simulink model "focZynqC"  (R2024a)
settings: Solver=ode45  StartTime=0.0  StopTime=10.0  RelTol=1e-3  EnableMultiTasking=on
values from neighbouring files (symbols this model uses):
  dataRange = Rotor velocity
                        radian/sec
                        800.0
                        -800.0
                    
                
                
                    
                        Phase current
                        Ampere
                        12.0
                        -12.0    [focZynqData.sldd]
  paramEncoderCalibrationDuration = 0.2
                
                    
                        Auto
                        
                        
                        -1.0
                        Simulink
                        Parameter
                        Default
                        
                            
                                0    [focZynqData.sldd]
  paramEncoderCalibrationMaxError = 0.0012566370614359172
                
                    
                        Auto
                        
                        
                        -1.0
                        Simulink
                        Parameter
                        Default
                        
                            
                                0    [focZynqData.sldd]
  paramEncoderCalibrationVoltage = 2.0
                
                    
                        Auto
                        
                        
                        -1.0
                        Simulink
                        Parameter
                        Default
                        
                            
                                0    [focZynqData.sldd]
  paramEncoderRotorPositionAtZeroCount = 0.0
                
                    
                        Auto
                        
                        
                        -1.0
                        Simulink
                        Parameter
                        Default
                        
                            
                                0    [focZynqData.sldd]
  paramOpenLoopVelocityAcceleration = 40.0
                
                    
                        Auto
                        
                        
                        -1.0
                        Simulink
                        Parameter
                        Default
                        
                            
                                0    [focZynqData.sldd]
  paramOpenLoopVelocityToVoltsBias = 0.4
                
                    
                        Auto
                        
                        
                        -1.0
                        Simulink
                        Parameter
                        Default
                        
                            
                                0    [focZynqData.sldd]
  paramOpenLoopVelocityToVoltsScalar = 0.04
                
                    
                        Auto
                        
                        
                        -1.0
                        Simulink
                        Parameter
                        Default
                        
                            
                                0    [focZynqData.sldd]
  paramVelocityControlI = 0.1
                
                    
                        Auto
                        
                        
                        -1.0
                        Simulink
                        Parameter
                        Default
                        
                            
                                0    [focZynqData.sldd]
  paramVelocityControlP = 0.02
                
                    
                        Auto
                        
                        
                        -1.0
                        Simulink
                        Parameter
                        Default
                        
                            
                                0    [focZynqData.sldd]
  paramVelocityControlSatCurrent = 4.0
                
                    
                        Auto
                        
                        
                        -1.0
                        Simulink
                        Parameter
                        Default
                        
                            
                                0    [focZynqData.sldd]
  pmsm = Dyno 1: BLY172D-24V-4000 Anaheim Automation
                BLY172D-24V-4000 Anaheim Automation
Phase A leads B leads C for counterclockwise rotation
-----------------------------------------------------
Phase A = Yellow
Phase B = Red
Phase C = Black
                
                    
                        Watt
                        Volt
                        rad/sec    [focZynqData.sldd]
  sampleTime = 4.0E-5
                0.001
                0.001
                4.0E-5
                2.0E-8
                4.0E-5
                0.001
                2.0E-8
                2.0E-8
                2.0E-8    [focZynqData.sldd]
libraries: simulink x2

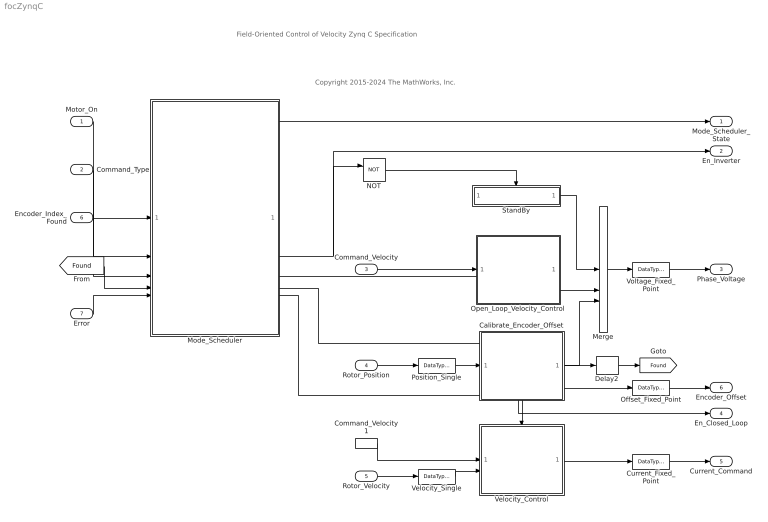
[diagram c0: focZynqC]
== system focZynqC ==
  note: Copyright 2015-2024 The MathWorks, Inc.
  note: Field-Oriented Control of Velocity Zynq C Specification
  Motor_On : Inport  OutDataTypeStr=boolean
  Command_Type : Inport  Port=2  OutDataTypeStr=Enum: commandTypeEnum
  Command_Velocity : Inport  Port=3
  Rotor_Position : Inport  Port=4  OutMin=0  OutMax=2*pi  OutDataTypeStr=fixdt(1,16,12)  SampleTime=sampleTime.VelocityControl
  Rotor_Velocity : Inport  Port=5  OutMin=dataRange.RotorVelocity.Min  OutMax=dataRange.RotorVelocity.Max  OutDataTypeStr=fixdt(1,16,5)
  Encoder_Index_Found : Inport  Port=6  OutDataTypeStr=boolean
  Error : Inport  Port=7  OutDataTypeStr=boolean
  Calibrate_Encoder_Offset : Subsystem
  Command_Velocity1 : InportShadow  Port=3
  Current_Fixed_Point : DataTypeConversion  OutMin=dataRange.PhaseCurrent.Min  OutMax=dataRange.PhaseCurrent.Max  OutDataTypeStr=fixdt(1,16,11)
  Delay2 : Delay  DelayLength=1
  Merge : Merge  Inputs=3
  Mode_Scheduler : Stateflow chart  TreatAsAtomicUnit=on
  NOT : Logic  Operator=NOT  IconShape=distinctive  AllPortsSameDT=off  OutDataTypeStr=boolean
  Offset_Fixed_Point : DataTypeConversion  OutMin=0  OutMax=2*pi  OutDataTypeStr=fixdt(1,16,12)
  Open_Loop_Velocity_Control : Subsystem  TreatAsAtomicUnit=on
  Position_Single : DataTypeConversion  OutDataTypeStr=single
  StandBy : Subsystem  Description=Stand By mode for controller outputs constant phase voltages.  TreatAsAtomicUnit=on
  Velocity_Control : Subsystem
  Velocity_Single : DataTypeConversion  OutDataTypeStr=single
  Voltage_Fixed_Point : DataTypeConversion  OutMin=dataRange.DqVoltage.Min  OutMax=dataRange.DqVoltage.Max  OutDataTypeStr=fixdt(1,16,11)
  Mode_Scheduler_State : Outport  VectorParamsAs1DForOutWhenUnconnected=off
  En_Inverter : Outport  Port=2  VectorParamsAs1DForOutWhenUnconnected=off
  Phase_Voltage : Outport  Port=3  VectorParamsAs1DForOutWhenUnconnected=off
  En_Closed_Loop : Outport  Port=4  VectorParamsAs1DForOutWhenUnconnected=off
  Current_Command : Outport  Port=5  VectorParamsAs1DForOutWhenUnconnected=off
  Encoder_Offset : Outport  Port=6  VectorParamsAs1DForOutWhenUnconnected=off
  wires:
  Rotor_Velocity/1 -> Velocity_Single/1
  Encoder_Index_Found/1 -> Mode_Scheduler/3(encoderIndexFound)
  Command_Velocity1/1 -> Velocity_Control/1(Velocity_Command)
  Command_Velocity/1 -> Open_Loop_Velocity_Control/1(Velocity_Command)
  [Found] -> Mode_Scheduler/4(encoderOffsetFound)
  Mode_Scheduler/4(" calibrateEncoder") -> Calibrate_Encoder_Offset/Enable
  Mode_Scheduler/1(mode) -> Mode_Scheduler_State/1
  Command_Type/1 -> Mode_Scheduler/2(commandType)
  Delay2/1 -> [Found]
  Error/1 -> Mode_Scheduler/5(error)
  Rotor_Position/1 -> Position_Single/1
  Calibrate_Encoder_Offset/3(Position_At_Zero_Count) -> Offset_Fixed_Point/1
  Calibrate_Encoder_Offset/2(Position_At_Zero_Count_Valid) -> Delay2/1
  Merge/1 -> Voltage_Fixed_Point/1
  Open_Loop_Velocity_Control/1(Phase_Voltage) -> Merge/2
  Calibrate_Encoder_Offset/1(Phase_Voltage) -> Merge/3
  Velocity_Control/1(Q_Current_Command) -> Current_Fixed_Point/1
  Motor_On/1 -> Mode_Scheduler/1(motorOn)
  Mode_Scheduler/3(" openLoop") -> Open_Loop_Velocity_Control/Enable
  Mode_Scheduler/5(" closedLoop") -> Velocity_Control/Enable, En_Closed_Loop/1
  Mode_Scheduler/2(" enableInverter") -> NOT/1, En_Inverter/1
  NOT/1 -> StandBy/Enable
  StandBy/1(Phase Voltage) -> Merge/1
  Voltage_Fixed_Point/1 -> Phase_Voltage/1
  Current_Fixed_Point/1 -> Current_Command/1
  Position_Single/1 -> Calibrate_Encoder_Offset/1(Rotor_Position)
  Velocity_Single/1 -> Velocity_Control/2(Velocity_Measured)
  Offset_Fixed_Point/1 -> Encoder_Offset/1

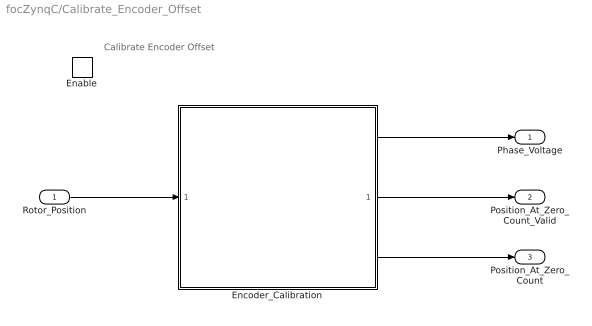
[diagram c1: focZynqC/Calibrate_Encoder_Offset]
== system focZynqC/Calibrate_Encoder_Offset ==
  note: Calibrate Encoder Offset
  Rotor_Position : Inport  PortDimensions=1  Interpolate=off
  Enable : EnablePort  StatesWhenEnabling=reset
  Encoder_Calibration : Subsystem
  Phase_Voltage : Outport  PortDimensions=3  InitialOutput=0  VectorParamsAs1DForOutWhenUnconnected=off
  Position_At_Zero_Count_Valid : Outport  Port=2  InitialOutput=0  VectorParamsAs1DForOutWhenUnconnected=off
  Position_At_Zero_Count : Outport  Port=3  InitialOutput=paramEncoderRotorPositionAtZeroCount  VectorParamsAs1DForOutWhenUnconnected=off
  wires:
  Encoder_Calibration/3(Position_At_Zero_Count) -> Position_At_Zero_Count/1
  Encoder_Calibration/2(Position_Valid) -> Position_At_Zero_Count_Valid/1
  Encoder_Calibration/1(Phase_Voltage) -> Phase_Voltage/1
  Rotor_Position/1 -> Encoder_Calibration/1(Rotor_Position)

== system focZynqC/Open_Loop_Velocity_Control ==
  note: Open Loop Velocity Control
  Velocity_Command : Inport
  Enable : EnablePort  StatesWhenEnabling=reset
  Open_Loop_Velocity_Control : Subsystem
  Phase_Voltage : Outport  VectorParamsAs1DForOutWhenUnconnected=off
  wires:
  Open_Loop_Velocity_Control/1(Phase_Voltage) -> Phase_Voltage/1  "phaseVoltage"
  Velocity_Command/1 -> Open_Loop_Velocity_Control/1(Velocity_Command)

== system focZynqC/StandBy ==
  note: Disabled
  Enable : EnablePort
  Constant : Constant  Value=[0 0 0]  OutDataTypeStr=Inherit: Inherit via back propagation
  Phase Voltage : Outport  InitialOutput=[0 0 0]  VectorParamsAs1DForOutWhenUnconnected=off
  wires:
  Constant/1 -> Phase Voltage/1

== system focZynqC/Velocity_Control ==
  note: Velocity Control
  Velocity_Command : Inport
  Velocity_Measured : Inport  Port=2
  Enable : EnablePort  StatesWhenEnabling=reset
  Velocity_Control : Subsystem
  Q_Current_Command : Outport  InitialOutput=0  VectorParamsAs1DForOutWhenUnconnected=off
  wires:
  Velocity_Command/1 -> Velocity_Control/1(Velocity_Command)
  Velocity_Measured/1 -> Velocity_Control/2(Velocity_Measured)  "rotorVelocity"
  Velocity_Control/1(Current) -> Q_Current_Command/1  "qCurrentCommand"

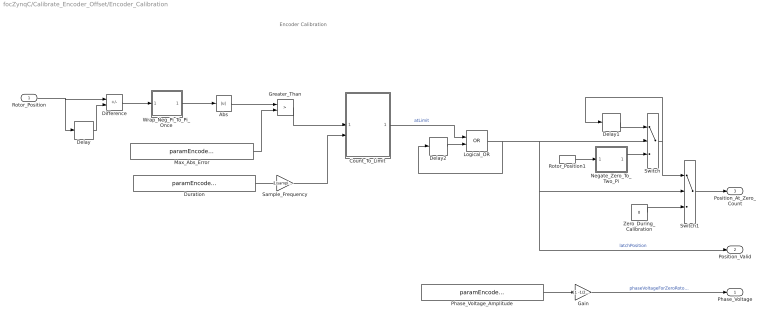
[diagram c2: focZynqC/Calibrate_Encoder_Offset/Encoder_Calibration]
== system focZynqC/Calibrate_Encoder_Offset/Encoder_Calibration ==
  note: Encoder Calibration
  Rotor_Position : Inport  OutMin=0  OutMax=2*pi  PortDimensions=1  SampleTime=sampleTime.EncoderCalibration  Interpolate=off
  Abs : Abs
  Count_To_Limit : Subsystem
  Delay : Delay  DelayLength=1
  Delay1 : Delay  DelayLength=1  InitialCondition=0
  Delay2 : Delay  DelayLength=1  InitialCondition=0
  Difference : Sum  Inputs=+-
  Duration : Constant  Value=paramEncoderCalibrationDuration  OutDataTypeStr=Inherit: Inherit via back propagation  SampleTime=-1
  Gain : Gain  Gain=[1 -1/2 -1/2]
  Greater_Than : RelationalOperator  Operator=>  OutDataTypeStr=boolean
  Logical_OR : Logic  Operator=OR  IconShape=distinctive  AllPortsSameDT=off  OutDataTypeStr=boolean
  Max_Abs_Error : Constant  Value=paramEncoderCalibrationMaxError  OutDataTypeStr=Inherit: Inherit via back propagation  SampleTime=-1
  Negate_Zero_To_Two_Pi : Subsystem
  Phase_Voltage_Amplitude : Constant  Value=paramEncoderCalibrationVoltage  OutDataTypeStr=Inherit: Inherit via back propagation  SampleTime=-1
  Rotor_Position1 : InportShadow  OutMin=0  OutMax=2*pi  PortDimensions=1  SampleTime=sampleTime.EncoderCalibration  Interpolate=off
  Sample_Frequency : Gain  Gain=1/sampleTime.EncoderCalibration
  Switch : Switch  Criteria=u2 ~= 0  Threshold=1
  Switch1 : Switch  Threshold=1
  Wrap_Neg_Pi_To_Pi_Once : Subsystem
  Zero_During_Calibration : Constant  Value=0  OutDataTypeStr=Inherit: Inherit via back propagation
  Phase_Voltage : Outport  SampleTime=sampleTime.EncoderCalibration  InitialOutput=0  VectorParamsAs1DForOutWhenUnconnected=off
  Position_Valid : Outport  Port=2  SampleTime=sampleTime.EncoderCalibration  InitialOutput=0  VectorParamsAs1DForOutWhenUnconnected=off
  Position_At_Zero_Count : Outport  Port=3  SampleTime=sampleTime.EncoderCalibration  InitialOutput=0  VectorParamsAs1DForOutWhenUnconnected=off
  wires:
  Greater_Than/1 -> Count_To_Limit/1(Reset)
  Gain/1 -> Phase_Voltage/1  "phaseVoltageForZeroRotorPosition"
  Phase_Voltage_Amplitude/1 -> Gain/1
  Duration/1 -> Sample_Frequency/1
  Difference/1 -> Wrap_Neg_Pi_To_Pi_Once/1(Position)
  Wrap_Neg_Pi_To_Pi_Once/1(Wrap) -> Abs/1
  Switch1/1 -> Position_At_Zero_Count/1
  Abs/1 -> Greater_Than/1
  Max_Abs_Error/1 -> Greater_Than/2
  Zero_During_Calibration/1 -> Switch1/3
  Logical_OR/1 -> Delay2/1, Position_Valid/1, Switch1/2, Switch/2  "latchPosition"
  Rotor_Position/1 -> Delay/1, Difference/1
  Switch/1 -> Switch1/1, Delay1/1
  Delay/1 -> Difference/2
  Rotor_Position1/1 -> Negate_Zero_To_Two_Pi/1(In)
  Delay1/1 -> Switch/1
  Negate_Zero_To_Two_Pi/1(Out) -> Switch/3
  Sample_Frequency/1 -> Count_To_Limit/2(Limit)
  Count_To_Limit/1(At_Limit) -> Logical_OR/1  "atLimit"
  Delay2/1 -> Logical_OR/2

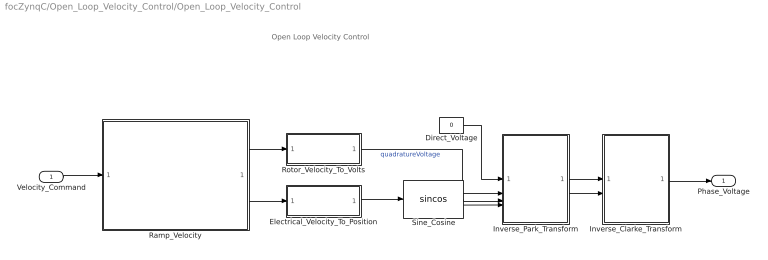
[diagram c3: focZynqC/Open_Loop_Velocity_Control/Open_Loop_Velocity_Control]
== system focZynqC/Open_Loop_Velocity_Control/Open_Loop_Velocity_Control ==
  note: Open Loop Velocity Control
  Velocity_Command : Inport  SampleTime=sampleTime.OpenLoopVelocityControl
  Direct_Voltage : Constant  Value=0  OutDataTypeStr=Inherit: Inherit via back propagation
  Electrical_Velocity_To_Position : Subsystem
  Inverse_Clarke_Transform : Subsystem  VariantControl=INVERSE_CLARKE_TRANSFORM
  Inverse_Park_Transform : Subsystem
  Ramp_Velocity : Subsystem
  Rotor_Velocity_To_Volts : Subsystem
  Sine_Cosine : Trigonometry  Operator=sincos
  Phase_Voltage : Outport  SampleTime=sampleTime.OpenLoopVelocityControl  VectorParamsAs1DForOutWhenUnconnected=off
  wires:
  Inverse_Clarke_Transform/1(ABC) -> Phase_Voltage/1
  Velocity_Command/1 -> Ramp_Velocity/1(Velocity_Command)
  Rotor_Velocity_To_Volts/1(V) -> Inverse_Park_Transform/2(Q)  "quadratureVoltage"
  Direct_Voltage/1 -> Inverse_Park_Transform/1(D)
  Inverse_Park_Transform/1(Alpha) -> Inverse_Clarke_Transform/1(Alpha)
  Inverse_Park_Transform/2(Beta) -> Inverse_Clarke_Transform/2(Beta)
  Ramp_Velocity/1(Rotor_Velocity) -> Rotor_Velocity_To_Volts/1(RV)
  Ramp_Velocity/2(Electrical_Velocity) -> Electrical_Velocity_To_Position/1(EV)
  Sine_Cosine/1 -> Inverse_Park_Transform/3(Sin_Coefficient1)
  Sine_Cosine/2 -> Inverse_Park_Transform/4(Cos_Coefficient1)
  Electrical_Velocity_To_Position/1(EP) -> Sine_Cosine/1

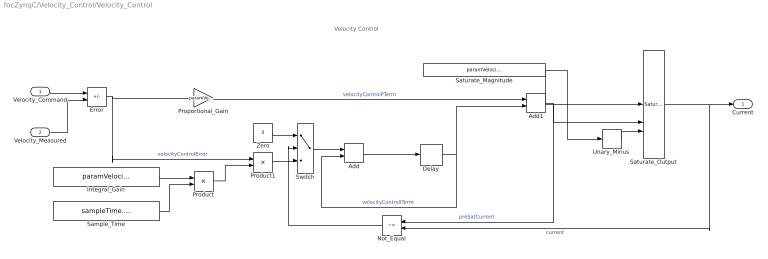
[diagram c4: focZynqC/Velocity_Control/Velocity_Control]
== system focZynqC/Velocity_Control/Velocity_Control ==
  note: Velocity Control
  Velocity_Command : Inport  SampleTime=sampleTime.VelocityControl
  Velocity_Measured : Inport  Port=2  SampleTime=sampleTime.VelocityControl
  Add : Sum
  Add1 : Sum
  Delay : Delay  DelayLength=1
  Error : Sum  Inputs=+-
  Integral_Gain : Constant  Value=paramVelocityControlI  OutDataTypeStr=Inherit: Inherit via back propagation
  Not_Equal : RelationalOperator  Operator=~=  OutDataTypeStr=boolean
  Product : Product
  Product1 : Product
  Proportional_Gain : Gain  Gain=paramVelocityControlP
  Sample_Time : Constant  Value=sampleTime.VelocityControl  OutDataTypeStr=Inherit: Inherit via back propagation
  Saturate_Magnitude : Constant  Value=paramVelocityControlSatCurrent  OutDataTypeStr=Inherit: Inherit via back propagation
  Saturate_Output : simulink/Discontinuities/Saturation Dynamic  OutMin=[]  OutMax=[]  OutDataTypeStr=Inherit: Same as second input  OutDataType=fixdt(1, 16)  OutScaling=2^-10  DoSatur=off
  Switch : Switch  Criteria=u2 ~= 0
  Unary_Minus : UnaryMinus
  Zero : Constant  Value=0  OutDataTypeStr=Inherit: Inherit via back propagation
  Current : Outport  SampleTime=sampleTime.VelocityControl  VectorParamsAs1DForOutWhenUnconnected=off
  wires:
  Add/1 -> Delay/1
  Product1/1 -> Switch/3
  Product/1 -> Product1/2
  Sample_Time/1 -> Product/2
  Integral_Gain/1 -> Product/1
  Unary_Minus/1 -> Saturate_Output/3
  Saturate_Magnitude/1 -> Unary_Minus/1, Saturate_Output/1
  Zero/1 -> Switch/1
  Switch/1 -> Add/1
  Not_Equal/1 -> Switch/2
  Saturate_Output/1 -> Not_Equal/2, Current/1  "current"
  Error/1 -> Product1/1, Proportional_Gain/1  "velocityControlError"
  Proportional_Gain/1 -> Add1/1  "velocityControlPTerm"
  Velocity_Command/1 -> Error/1
  Add1/1 -> Saturate_Output/2, Not_Equal/1  "preSatCurrent"
  Delay/1 -> Add1/2, Add/2  "velocityControlITerm"
  Velocity_Measured/1 -> Error/2

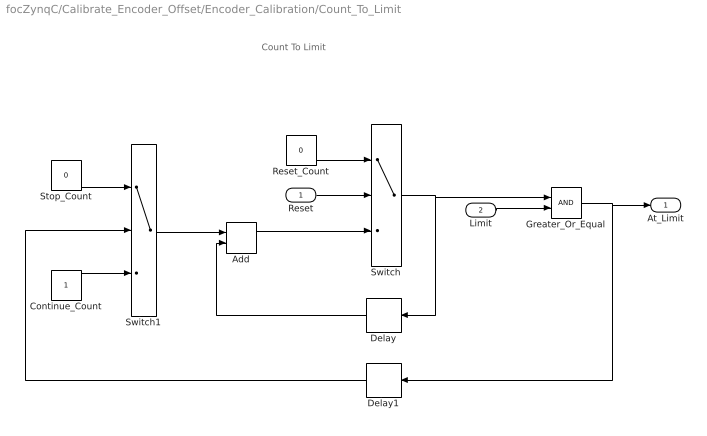
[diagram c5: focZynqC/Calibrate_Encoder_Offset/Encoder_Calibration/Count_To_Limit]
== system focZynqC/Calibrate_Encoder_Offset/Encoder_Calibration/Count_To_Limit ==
  note: Count To Limit
  Reset : Inport
  Limit : Inport  Port=2
  Add : Sum
  Continue_Count : Constant  OutDataTypeStr=Inherit: Inherit via back propagation
  Delay : Delay  DelayLength=1  InitialCondition=0
  Delay1 : Delay  DelayLength=1  InitialCondition=0
  Greater_Or_Equal : RelationalOperator  OutDataTypeStr=boolean
  Reset_Count : Constant  Value=0  OutDataTypeStr=Inherit: Inherit via back propagation
  Stop_Count : Constant  Value=0  OutDataTypeStr=Inherit: Inherit via back propagation
  Switch : Switch  Threshold=1
  Switch1 : Switch  Threshold=1
  At_Limit : Outport  VectorParamsAs1DForOutWhenUnconnected=off
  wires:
  Add/1 -> Switch/3
  Reset_Count/1 -> Switch/1
  Reset/1 -> Switch/2
  Delay/1 -> Add/2
  Greater_Or_Equal/1 -> At_Limit/1, Delay1/1
  Stop_Count/1 -> Switch1/1
  Switch/1 -> Greater_Or_Equal/1, Delay/1
  Continue_Count/1 -> Switch1/3
  Switch1/1 -> Add/1
  Limit/1 -> Greater_Or_Equal/2
  Delay1/1 -> Switch1/2

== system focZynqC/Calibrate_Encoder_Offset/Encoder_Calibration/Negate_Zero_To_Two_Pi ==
  note: Negate Zero To Two Pi
  In : Inport
  Input_Range : SignalSpecification  OutMin=0  OutMax=2*pi
  Subtract : Sum  Inputs=+-  OutDataTypeStr=Inherit: Inherit via back propagation
  Two_Pi : Constant  Value=2*pi  OutDataTypeStr=Inherit: Inherit via back propagation
  Out : Outport  VectorParamsAs1DForOutWhenUnconnected=off
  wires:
  Subtract/1 -> Out/1  "negativeIn"
  In/1 -> Input_Range/1
  Two_Pi/1 -> Subtract/1
  Input_Range/1 -> Subtract/2

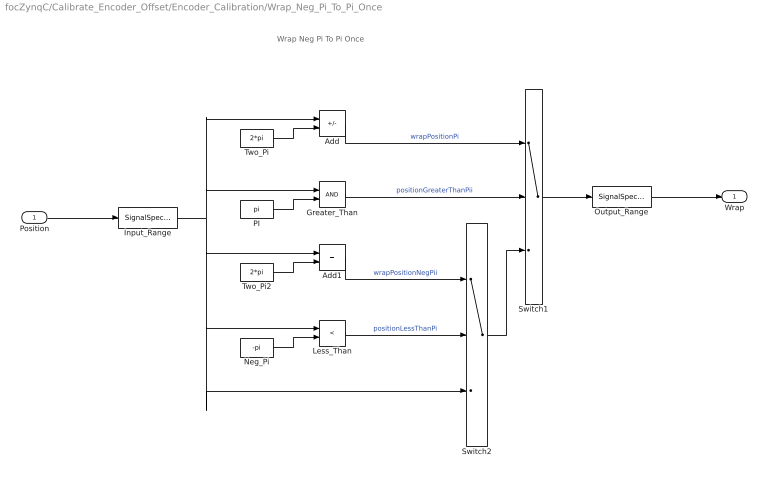
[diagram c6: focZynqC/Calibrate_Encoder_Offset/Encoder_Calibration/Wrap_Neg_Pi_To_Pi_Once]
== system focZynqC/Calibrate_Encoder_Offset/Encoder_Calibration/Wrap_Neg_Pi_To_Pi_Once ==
  note: Wrap Neg Pi To Pi Once
  Position : Inport
  Add : Sum  Inputs=+-  OutDataTypeStr=Inherit: Inherit via back propagation
  Add1 : Sum
  Greater_Than : RelationalOperator  OutDataTypeStr=boolean
  Input_Range : SignalSpecification  OutMin=-4*pi  OutMax=4*pi
  Less_Than : RelationalOperator  Operator=<  OutDataTypeStr=boolean
  Neg_Pi : Constant  Value=-pi  OutDataTypeStr=Inherit: Inherit via back propagation
  Output_Range : SignalSpecification  OutMin=-pi  OutMax=pi
  PI : Constant  Value=pi  OutDataTypeStr=Inherit: Inherit via back propagation
  Switch1 : Switch  Criteria=u2 ~= 0
  Switch2 : Switch  Criteria=u2 ~= 0
  Two_Pi : Constant  Value=2*pi  OutDataTypeStr=Inherit: Inherit via back propagation
  Two_Pi2 : Constant  Value=2*pi  OutDataTypeStr=Inherit: Inherit via back propagation
  Wrap : Outport  VectorParamsAs1DForOutWhenUnconnected=off
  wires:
  Position/1 -> Input_Range/1
  PI/1 -> Greater_Than/2
  Neg_Pi/1 -> Less_Than/2
  Greater_Than/1 -> Switch1/2  "positionGreaterThanPii"
  Two_Pi/1 -> Add/2
  Add/1 -> Switch1/1  "wrapPositionPi"
  Less_Than/1 -> Switch2/2  "positionLessThanPi"
  Switch2/1 -> Switch1/3
  Two_Pi2/1 -> Add1/2
  Add1/1 -> Switch2/1  "wrapPositionNegPii"
  Switch1/1 -> Output_Range/1
  Output_Range/1 -> Wrap/1
  Input_Range/1 -> Less_Than/1, Switch2/3, Add1/1, Add/1, Greater_Than/1

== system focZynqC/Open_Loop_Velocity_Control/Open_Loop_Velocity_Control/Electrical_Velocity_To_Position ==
  note: Electrical Velocity To Position
  EV : Inport
  Add : Sum
  Delay : Delay  DelayLength=1
  Gain : Gain  Gain=sampleTime.OpenLoopVelocityControl  OutDataTypeStr=Inherit: Inherit via back propagation
  Mod_Two_Pi_Once : Subsystem
  EP : Outport  VectorParamsAs1DForOutWhenUnconnected=off
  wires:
  Delay/1 -> Add/2, EP/1
  Gain/1 -> Add/1
  EV/1 -> Gain/1
  Mod_Two_Pi_Once/1(Mod_X_Two_Pi) -> Delay/1
  Add/1 -> Mod_Two_Pi_Once/1(X)

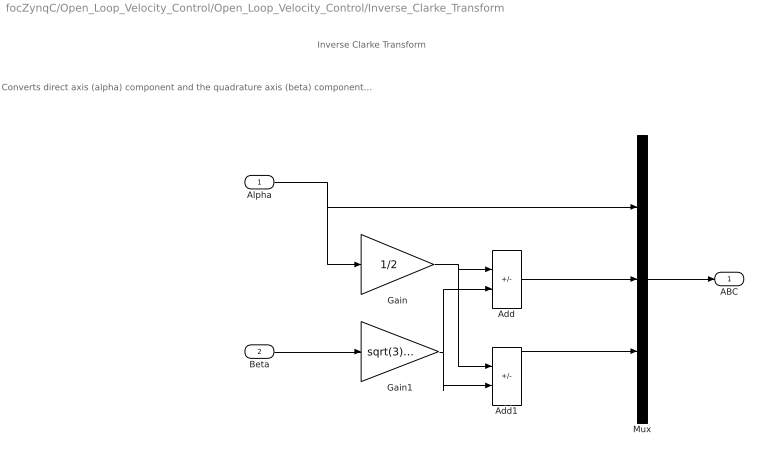
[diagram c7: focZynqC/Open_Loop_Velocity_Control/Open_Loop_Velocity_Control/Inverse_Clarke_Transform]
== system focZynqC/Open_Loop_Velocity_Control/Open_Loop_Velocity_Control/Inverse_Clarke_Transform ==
  note: Inverse Clarke Transform
  note: Converts direct axis (alpha) component and the quadrature axis (beta) component to balanced three-phase quantities The alpha and beta components are dependent on time and speed.
  Alpha : Inport
  Beta : Inport  Port=2
  Add : Sum  Inputs=-+
  Add1 : Sum  Inputs=--
  Gain : Gain  Gain=1/2
  Gain1 : Gain  Gain=sqrt(3)/2
  Mux : Mux  Inputs=3
  ABC : Outport  VectorParamsAs1DForOutWhenUnconnected=off
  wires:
  Gain/1 -> Add1/1, Add/1
  Gain1/1 -> Add1/2, Add/2
  Add/1 -> Mux/2
  Add1/1 -> Mux/3
  Beta/1 -> Gain1/1
  Alpha/1 -> Mux/1, Gain/1
  Mux/1 -> ABC/1

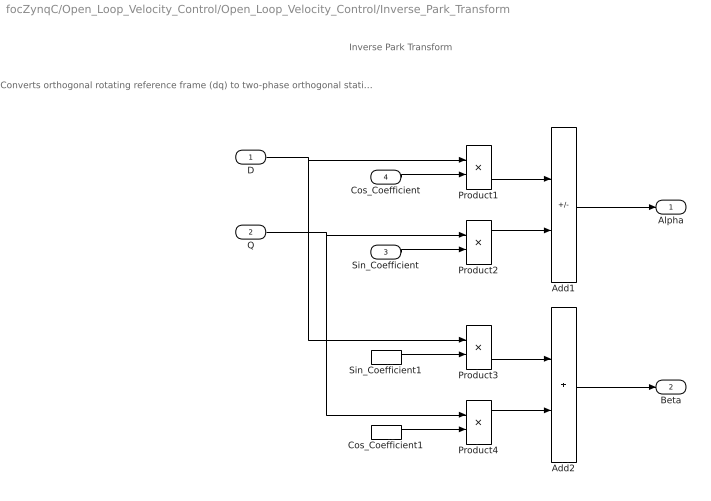
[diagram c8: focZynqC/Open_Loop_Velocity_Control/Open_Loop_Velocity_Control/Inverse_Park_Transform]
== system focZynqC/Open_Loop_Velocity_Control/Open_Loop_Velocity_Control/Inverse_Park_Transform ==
  note: Inverse Park Transform
  note: Converts orthogonal rotating reference frame (dq) to two-phase orthogonal stationary reference frame (alpha, beta)
  D : Inport
  Q : Inport  Port=2
  Sin_Coefficient : Inport  Port=3
  Cos_Coefficient : Inport  Port=4
  Add1 : Sum  Inputs=+-
  Add2 : Sum
  Cos_Coefficient1 : InportShadow  Port=4
  Product{1..4} (4 alike) : Product  RndMeth=Simplest
  Sin_Coefficient1 : InportShadow  Port=3
  Alpha : Outport  VectorParamsAs1DForOutWhenUnconnected=off
  Beta : Outport  Port=2  VectorParamsAs1DForOutWhenUnconnected=off
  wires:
  Add2/1 -> Beta/1
  Add1/1 -> Alpha/1
  Product3/1 -> Add2/1
  Product4/1 -> Add2/2
  Product1/1 -> Add1/1
  Product2/1 -> Add1/2
  Cos_Coefficient1/1 -> Product4/2
  Sin_Coefficient/1 -> Product2/2
  D/1 -> Product3/1, Product1/1
  Q/1 -> Product2/1, Product4/1
  Sin_Coefficient1/1 -> Product3/2
  Cos_Coefficient/1 -> Product1/2

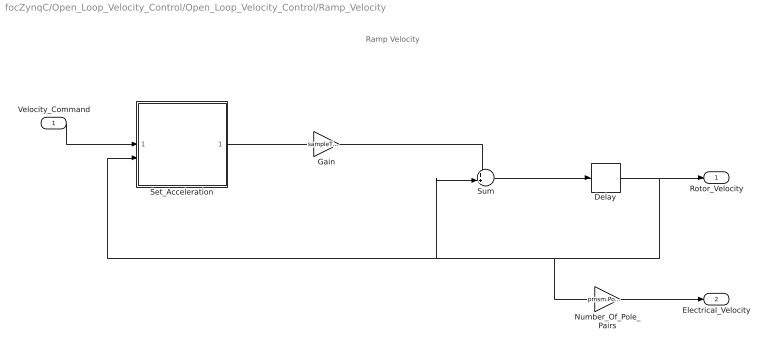
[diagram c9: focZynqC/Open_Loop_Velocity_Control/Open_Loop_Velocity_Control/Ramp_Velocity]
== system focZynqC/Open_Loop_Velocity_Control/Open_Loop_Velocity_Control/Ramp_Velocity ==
  note: Ramp Velocity
  Velocity_Command : Inport
  Delay : Delay  DelayLength=1
  Gain : Gain  Gain=sampleTime.OpenLoopVelocityControl
  Number_Of_Pole_Pairs : Gain  Gain=pmsm.PolePairs
  Set_Acceleration : Subsystem
  Sum : Sum  Inputs=++|  SaturateOnIntegerOverflow=on
  Rotor_Velocity : Outport  VectorParamsAs1DForOutWhenUnconnected=off
  Electrical_Velocity : Outport  Port=2  VectorParamsAs1DForOutWhenUnconnected=off
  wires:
  Number_Of_Pole_Pairs/1 -> Electrical_Velocity/1
  Set_Acceleration/1(A) -> Gain/1
  Velocity_Command/1 -> Set_Acceleration/1(V_Target)
  Gain/1 -> Sum/1
  Delay/1 -> Set_Acceleration/2(V_Current), Sum/2, Number_Of_Pole_Pairs/1, Rotor_Velocity/1
  Sum/1 -> Delay/1

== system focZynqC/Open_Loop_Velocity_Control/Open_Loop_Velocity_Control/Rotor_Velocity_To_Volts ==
  note: Rotor Velocity To Volts
  RV : Inport
  Abs : Abs
  Add : Sum
  Frequency_To_Voltage : Gain  Gain=paramOpenLoopVelocityToVoltsScalar
  Voltage_Bias : Constant  Value=paramOpenLoopVelocityToVoltsBias  OutDataTypeStr=Inherit: Inherit via back propagation  SampleTime=-1
  V : Outport  VectorParamsAs1DForOutWhenUnconnected=off
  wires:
  RV/1 -> Abs/1
  Abs/1 -> Frequency_To_Voltage/1
  Frequency_To_Voltage/1 -> Add/2
  Add/1 -> V/1
  Voltage_Bias/1 -> Add/1

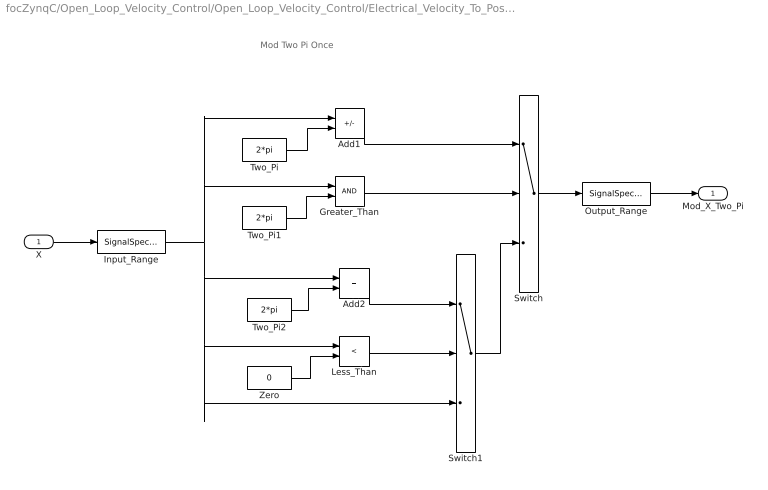
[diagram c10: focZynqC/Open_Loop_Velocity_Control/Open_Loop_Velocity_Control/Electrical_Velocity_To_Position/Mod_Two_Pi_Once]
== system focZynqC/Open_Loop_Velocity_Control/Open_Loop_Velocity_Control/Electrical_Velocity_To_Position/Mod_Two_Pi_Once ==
  note: Mod Two Pi Once
  X : Inport
  Add1 : Sum  Inputs=+-
  Add2 : Sum
  Greater_Than : RelationalOperator  OutDataTypeStr=boolean
  Input_Range : SignalSpecification  OutMin=-4*pi  OutMax=4*pi
  Less_Than : RelationalOperator  Operator=<  OutDataTypeStr=boolean
  Output_Range : SignalSpecification  OutMin=0  OutMax=2*pi
  Switch : Switch  Criteria=u2 ~= 0
  Switch1 : Switch  Criteria=u2 ~= 0
  Two_Pi : Constant  Value=2*pi  OutDataTypeStr=Inherit: Inherit via back propagation
  Two_Pi1 : Constant  Value=2*pi  OutDataTypeStr=Inherit: Inherit via back propagation
  Two_Pi2 : Constant  Value=2*pi  OutDataTypeStr=Inherit: Inherit via back propagation
  Zero : Constant  Value=0  OutDataTypeStr=Inherit: Inherit via back propagation
  Mod_X_Two_Pi : Outport  VectorParamsAs1DForOutWhenUnconnected=off
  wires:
  Input_Range/1 -> Switch1/3, Less_Than/1, Add2/1, Greater_Than/1, Add1/1
  Switch/1 -> Output_Range/1
  X/1 -> Input_Range/1
  Greater_Than/1 -> Switch/2
  Add1/1 -> Switch/1
  Two_Pi/1 -> Add1/2
  Two_Pi1/1 -> Greater_Than/2
  Switch1/1 -> Switch/3
  Less_Than/1 -> Switch1/2
  Add2/1 -> Switch1/1
  Two_Pi2/1 -> Add2/2
  Zero/1 -> Less_Than/2
  Output_Range/1 -> Mod_X_Two_Pi/1

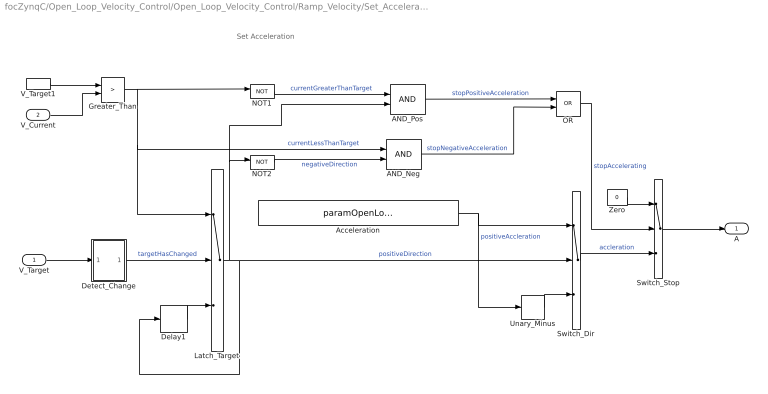
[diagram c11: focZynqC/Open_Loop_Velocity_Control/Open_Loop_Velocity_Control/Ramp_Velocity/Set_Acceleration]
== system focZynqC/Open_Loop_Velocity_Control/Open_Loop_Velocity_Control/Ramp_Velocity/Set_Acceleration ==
  note: Set Acceleration
  V_Target : Inport
  V_Current : Inport  Port=2
  AND_Neg : Logic  IconShape=distinctive  AllPortsSameDT=off  OutDataTypeStr=boolean
  AND_Pos : Logic  IconShape=distinctive  AllPortsSameDT=off  OutDataTypeStr=boolean
  Acceleration : Constant  Value=paramOpenLoopVelocityAcceleration  OutDataTypeStr=Inherit: Inherit via back propagation  SampleTime=-1
  Delay1 : Delay  DelayLength=1
  Detect_Change : Subsystem
  Greater_Than : RelationalOperator  Operator=>  OutDataTypeStr=boolean
  Latch_Target : Switch  Criteria=u2 ~= 0
  NOT1 : Logic  Operator=NOT  IconShape=distinctive  AllPortsSameDT=off  OutDataTypeStr=boolean
  NOT2 : Logic  Operator=NOT  IconShape=distinctive  AllPortsSameDT=off  OutDataTypeStr=boolean
  OR : Logic  Operator=OR  IconShape=distinctive  AllPortsSameDT=off  OutDataTypeStr=boolean
  Switch_Dir : Switch  Criteria=u2 > Threshold
  Switch_Stop : Switch  Criteria=u2 ~= 0
  Unary_Minus : UnaryMinus
  V_Target1 : InportShadow
  Zero : Constant  Value=0  OutDataTypeStr=Inherit: Inherit via back propagation  SampleTime=-1
  A : Outport  VectorParamsAs1DForOutWhenUnconnected=off
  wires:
  Latch_Target/1 -> AND_Pos/2, NOT2/1, Switch_Dir/2, Delay1/1  "positiveDirection"
  Greater_Than/1 -> NOT1/1, Latch_Target/1, AND_Neg/1  "currentLessThanTarget"
  Delay1/1 -> Latch_Target/3
  V_Current/1 -> Greater_Than/2
  V_Target1/1 -> Greater_Than/1
  V_Target/1 -> Detect_Change/1(X)
  Detect_Change/1(Y) -> Latch_Target/2  "targetHasChanged"
  Unary_Minus/1 -> Switch_Dir/3
  Acceleration/1 -> Unary_Minus/1, Switch_Dir/1  "positiveAccleration"
  Switch_Stop/1 -> A/1
  Switch_Dir/1 -> Switch_Stop/3  "accleration"
  Zero/1 -> Switch_Stop/1
  NOT1/1 -> AND_Pos/1  "currentGreaterThanTarget"
  AND_Pos/1 -> OR/1  "stopPositiveAcceleration"
  OR/1 -> Switch_Stop/2  "stopAccelerating"
  NOT2/1 -> AND_Neg/2  "negativeDirection"
  AND_Neg/1 -> OR/2  "stopNegativeAcceleration"

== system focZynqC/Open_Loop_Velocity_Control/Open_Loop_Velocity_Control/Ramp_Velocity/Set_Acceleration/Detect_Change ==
  note: Detect Change
  X : Inport
  Add : Sum  Inputs=+-
  Delay : Delay  DelayLength=1
  Not_Equal_Zero : simulink/Logic and Bit Operations/Compare To Zero  relop=~=  OutDataTypeStr=boolean
  Y : Outport  VectorParamsAs1DForOutWhenUnconnected=off
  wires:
  X/1 -> Delay/1, Add/1
  Not_Equal_Zero/1 -> Y/1
  Add/1 -> Not_Equal_Zero/1
  Delay/1 -> Add/2

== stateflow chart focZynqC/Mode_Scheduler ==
  state Mode Scheduler [group]
  state Enable_Inverter
    state Open_Loop
      state Open_Loop_Command
      state Find_Encoder_Index
    state Calibrate_Encoder_Offset
    state Closed_Loop
    (junction 378) -> Open_Loop_Command : [commandType == ...  commandTypeEnum.OpenLoopVelocity]
    (junction 378) -> (junction 624)
    Open_Loop_Command -> (junction 624) : [commandType ~= ...  commandTypeEnum.OpenLoopVelocity]
    (junction 624) -> (junction 619)
    (junction 619) -> (junction 638) : [(commandType == ...   commandTypeEnum.CalibrateEncoder) ...  || (paramEncoderCalibrateAtStartup ...      && ~encoderOffsetFound) ]
    (junction 638) -> Find_Encoder_Index : [~encoderIndexFound]
    (junction 638) -> (junction 640)
    (junction 619) -> (junction 604)
    Find_Encoder_Index -> Calibrate_Encoder_Offset : [encoderIndexFound]
    (junction 640) -> Calibrate_Encoder_Offset
    Calibrate_Encoder_Offset -> (junction 604) : [(commandType ~= ...   commandTypeEnum.CalibrateEncoder) ...   && encoderOffsetFound]
    (junction 604) -> (junction 232)
    (junction 232) -> Closed_Loop : [commandType == ...  commandTypeEnum.Velocity]
    (junction 232) -> (junction 627)
    Closed_Loop -> (junction 627) : [commandType ~= ...  commandTypeEnum.Velocity]
  state Stand_By
  state Error
  (default) -> Stand_By
  Stand_By -> (junction 378) : [motorOn]
  Enable_Inverter -> Stand_By : [~motorOn]
  Error -> Stand_By : [~motorOn]
  Enable_Inverter -> Error : [error]
  (junction 627) -> Error
  data: mode output Enum: modeSchedulerEnum; enableInverter output boolean; motorOn input; commandType input; encoderIndexFound input; openLoop output boolean; calibrateEncoder output boolean; closedLoop output boolean; encoderOffsetFound input; error input; paramEncoderCalibrateAtStartup parameter boolean
